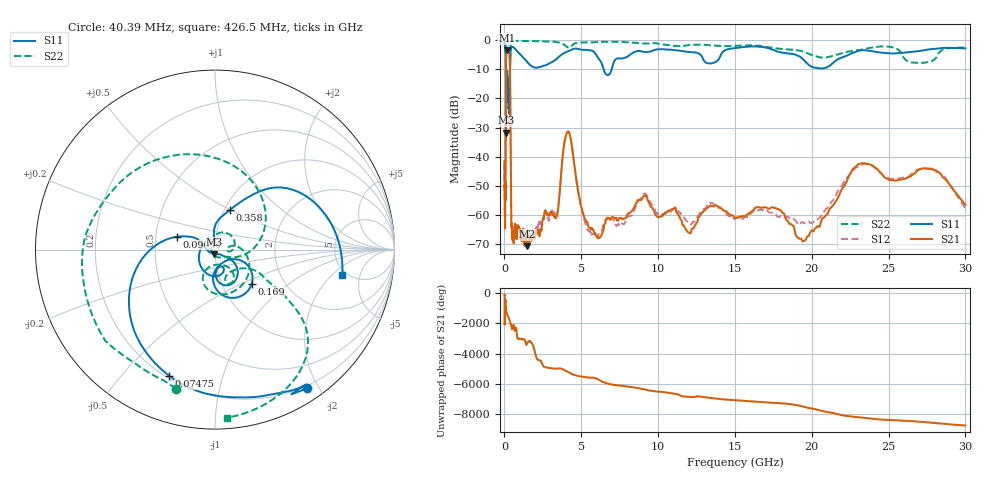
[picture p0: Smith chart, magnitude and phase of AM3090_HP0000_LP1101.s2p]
! Date/Time: Thu, Feb 28, 2019 1:53 PM
! Network Analyzer: Agilent Technologies E8364B Rev: A.07.50.67
! Sweep from 0.010 to 30.000 GHz, 1601 Points, Sweep Type: LOG
! Power Supply: 5.023 V, 0.002 A
# Hz S DB R 50
!freq MagS11 AngS11 MagS21 AngS21 MagS12 AngS12 MagS22 AngS22
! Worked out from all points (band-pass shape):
!   1601 points, 10 MHz to 30 GHz, reference 50 ohm
!   highest |S21| = -3.55 dB at 156 MHz (marker M1); lowest = -70.7 dB at 1.49 GHz (marker M2)
!   |S21| within 3 dB of the highest: 100.1 MHz to 343.7 MHz (243.6 MHz wide, 110 % of centre)
!   lowest |S11| = -31.8 dB at 97.94 MHz (marker M3), VSWR 1.05, Z = 49.3 - j2.46 ohm
!   |S11| at or under -10 dB: 88.93 MHz to 369.5 MHz (280.6 MHz wide, 122 % of centre); 6.455 GHz to 6.98 GHz (524.4 MHz wide, 7.81 % of centre)
!   |S22| runs from -33.9 to -0.1 dB; largest |S21 - S12| = 0.014
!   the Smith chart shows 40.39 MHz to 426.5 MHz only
!   S11 on the Smith chart (normalised r, x): 40.39 MHz: 0.17, -1.86; 74.75 MHz: 0.21, -0.68; 90.41 MHz: 0.64, +0.10; 169 MHz: 1.37, -0.57; 358 MHz: 1.06, +0.49; 426.5 MHz: 4.57, -2.71
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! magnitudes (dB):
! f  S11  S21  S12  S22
! 10 MHz  -0.2  -41.6  -42.2  -0.7
! 38.04 MHz  -0.5  -61.5  -61.0  -1.7
! 40.39 MHz  -0.7  -60.6  -61.2  -1.9
! 74.75 MHz  -2.5  -44.1  -43.8  -4.4
! 90.41 MHz  -13.0  -13.6  -13.6  -13.4
! 97.94 MHz  -31.8  -7.2  -7.2  -33.4
! 144.7 MHz  -19.2  -3.6  -3.6  -22.2
! 156 MHz  -13.6  -3.5  -3.5  -17.1
! 169 MHz  -11.1  -3.6  -3.6  -13.5
! 314.3 MHz  -25.2  -4.8  -4.7  -15.5
! 358 MHz  -12.6  -8.7  -8.7  -8.5
! 426.5 MHz  -2.8  -54.1  -52.6  -0.6
! 550.5 MHz  -2.4  -67.2  -65.1  -0.2
! 1.49 GHz  -7.6  -70.7  -68.9  -0.3
! 2.084 GHz  -9.5  -65.7  -64.0  -0.4
! 3.402 GHz  -6.4  -60.6  -60.2  -0.7
! 4.115 GHz  -3.9  -31.4  -31.4  -2.5
! 5.501 GHz  -3.4  -64.3  -65.6  -0.8
! 7.926 GHz  -5.9  -61.0  -61.6  -0.7
! 19.7 GHz  -8.0  -67.4  -62.5  -4.5
! 23.48 GHz  -3.5  -42.3  -42.4  -3.0
! 30 GHz  -2.8  -56.5  -57.6  -2.5
